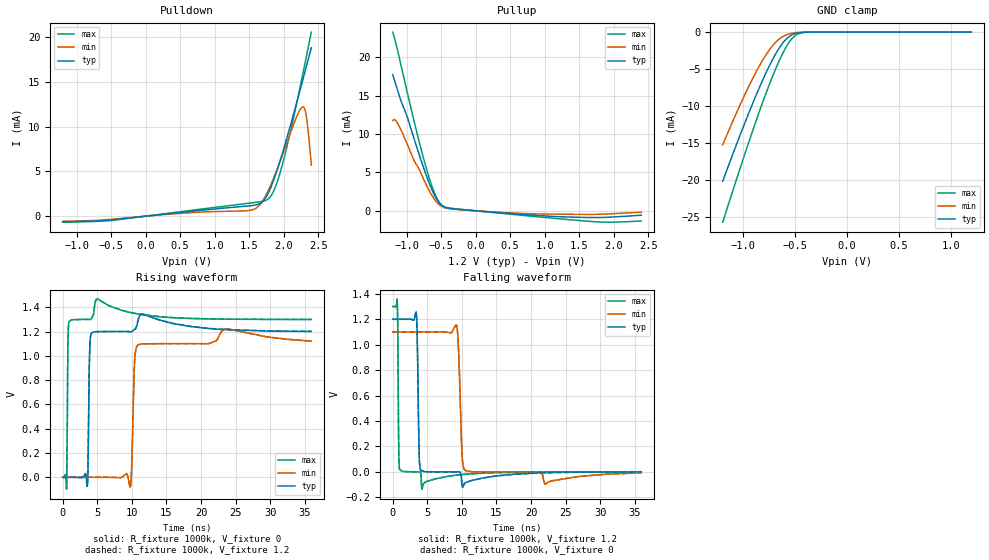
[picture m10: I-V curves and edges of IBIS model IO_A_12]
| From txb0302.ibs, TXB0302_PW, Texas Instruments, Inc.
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[Model]   IO_A_12
Model_type  3-state
Enable   Active-High
Vref =   0
Rref =   1000k
Cref =   50p
Vmeas =   0.6
| variable   typ   min   max
C_comp   3.49pF   3.27pF   3.66pF
| C_pullup   3.74pF   3.34pF   3.97pF
| C_pulldown   3.72pF   3.34pF   3.89pF
| C_tri-state   3.49pF   3.27pF   3.66pF
[Temperature Range]   40   100   -40
| Ambient temperature   25   85   -40
[Voltage range]   1.2   1.1   1.3
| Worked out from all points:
|   slope of the pulldown table from 0 to 0.18 V, typ, clamps not added: 1.19 kohm
|   slope of the pullup table from 0 to 0.18 V, typ, clamps not added: 1.36 kohm
|   GND clamp passes 1 mA (typ) near -0.59 V on its own axis
|   rising waveform, R_fixture 1000k, V_fixture 0: 20-80 % time 170ps typ, 302ps min, 102ps max; typ from 0 V to 1.2 V
|   falling waveform, R_fixture 1000k, V_fixture 1.2: 20-80 % time 206ps typ, 384ps min, 111ps max; typ from 1.2 V to 0.001 V
|   rising waveform, R_fixture 1000k, V_fixture 1.2: 20-80 % time 170ps typ, 303ps min, 102ps max; typ from 0.001 V to 1.2 V
|   falling waveform, R_fixture 1000k, V_fixture 0: 20-80 % time 206ps typ, 385ps min, 111ps max; typ from 1.2 V to 0 V
[GND Clamp]
| IO_A_12
|   Voltage   I(typ)   I(min)   I(max)
-1.2V     -20.17mA   -15.23mA   -25.71mA
-1.07V    -15.31mA   -11.02mA   -20.05mA
-960mV    -11.36mA   -7.676mA   -15.38mA
-865mV    -8.125mA   -5.054mA   -11.49mA
-785mV    -5.598mA   -3.138mA   -8.387mA
-705mV    -3.354mA   -1.626mA   -5.519mA
-630mV    -1.664mA   -696.5uA   -3.14mA
-565mV    -678.3uA   -271.2uA   -1.498mA
-505mV    -217.6uA   -92.4uA    -530uA
-450mV    -60.83uA   -27.6uA    -139.8uA
-365mV    -6.097uA   -3.22uA    -9.086uA
1.2V      188.6pA    17.64nA    18.68pA
[Pulldown]
| IO_A_12
|   Voltage   I(typ)   I(min)   I(max)
-1.2V     -625uA     -574.3uA   -672.8uA
-490mV    -412.4uA   -345.2uA   -476.2uA
1.505V    1.157mA    638.5uA    1.458mA
1.645V    1.372mA    1.202mA    1.593mA
1.775V    2.554mA    2.848mA    1.923mA
1.865V    4.251mA    4.459mA    2.98mA
1.965V    6.623mA    6.481mA    5.318mA
2.18V     12.46mA    10.97mA    12.33mA
2.27V     15.05mA    12.22mA    15.63mA
2.305V    16.06mA    11.97mA    16.95mA
2.33V     16.79mA    11.06mA    17.89mA
2.4V      18.83mA    5.724mA    20.58mA
[Pullup]
| IO_A_12
|   Voltage   I(typ)   I(min)   I(max)
-1.2V     17.76mA    11.76mA    23.31mA
-1.165V   16.75mA    11.84mA    22.21mA
-1.11V    15.16mA    11.1mA     20.16mA
-995mV    12.38mA    8.797mA    15.66mA
-875mV    8.963mA    6.299mA    11.11mA
-715mV    4.655mA    3.409mA    5.594mA
-585mV    1.873mA    1.367mA    2.106mA
-480mV    653.4uA    516.9uA    678.3uA
-295mV    225.5uA    188.7uA    266.9uA
1.175V    -755.5uA   -439.1uA   -1.013mA
1.84V     -865.1uA   -440.6uA   -1.479mA
2.4V      -573.8uA   -201.8uA   -1.327mA
[Ramp]
| IO_A_12
| variable   typ   min   max
dV/dt_r   0.85/2.39E-10   0.78/3.86E-10   0.94/1.46E-10
dV/dt_f   0.83/2.59E-10   0.75/4.53E-10   0.89/1.52E-10
R_load = 1000k
[Rising Waveform]
| IO_A_12
R_fixture =   1000k
C_fixture =   0
L_fixture =   0
V_fixture =   0
V_fixture_min = 0
V_fixture_max = 0
|   Time   V(typ)   V(min)   V(max)
0s        354nV      2.094uV    36.74nV
557ps     315.8nV    2.094uV    -97.53mV
853ps     98.54nV    2.094uV    1.262V
3.533ns   -75.7mV    2.023uV    1.3V
3.957ns   1.119V     1.896uV    1.298V
4.893ns   1.199V     3.631uV    1.467V
9.805ns   1.198V     -76.96mV   1.356V
10.38ns   1.217V     937.1mV    1.349V
10.88ns   1.291V     1.089V     1.344V
35.95ns   1.2V       1.12V      1.299V
[Falling Waveform]
| IO_A_12
R_fixture =   1000k
C_fixture =   0
L_fixture =   0
V_fixture =   1.2
V_fixture_min = 1.1
V_fixture_max = 1.3
|   Time   V(typ)   V(min)   V(max)
0s        1.2V       1.1V       1.3V
645ps     1.2V       1.1V       1.348V
949ps     1.2V       1.1V       33.34mV
3.405ns   1.257V     1.1V       66.36uV
3.837ns   119.4mV    1.1V       461.7uV
4.221ns   9.268mV    1.1V       -135.2mV
9.245ns   56.63uV    1.148V     -24.94mV
10.04ns   -114.2mV   120.7mV    -20.31mV
10.52ns   -83.51mV   10.88mV    -17.93mV
35.95ns   1.027mV    -6.454mV   1.269mV
[Rising Waveform]
| IO_A_12
R_fixture =   1000k
C_fixture =   0
L_fixture =   0
V_fixture =   1.2
V_fixture_min = 1.1
V_fixture_max = 1.3
|   Time   V(typ)   V(min)   V(max)
0s        1.421mV    1.618mV    1.31mV
557ps     1.421mV    1.618mV    -96.2mV
853ps     1.42mV     1.618mV    1.262V
3.533ns   -74.18mV   1.618mV    1.3V
3.957ns   1.119V     1.617mV    1.298V
4.893ns   1.199V     1.619mV    1.467V
9.805ns   1.198V     -75.03mV   1.357V
10.38ns   1.217V     937.9mV    1.35V
10.88ns   1.291V     1.089V     1.345V
35.95ns   1.202V     1.122V     1.3V
[Falling Waveform]
| IO_A_12
R_fixture =   1000k
C_fixture =   0
L_fixture =   0
V_fixture =   0
V_fixture_min = 0
V_fixture_max = 0
|   Time   V(typ)   V(min)   V(max)
0s        1.198V     1.098V     1.299V
645ps     1.198V     1.098V     1.346V
949ps     1.198V     1.098V     33.22mV
3.405ns   1.255V     1.098V     39.26uV
3.837ns   118.9mV    1.098V     436.4uV
4.221ns   9.225mV    1.098V     -135.5mV
9.245ns   27.76uV    1.146V     -25.93mV
10.04ns   -114.3mV   120mV      -21.35mV
10.52ns   -83.65mV   10.81mV    -19.01mV
35.95ns   -386uV     -7.912mV   -40.99uV
